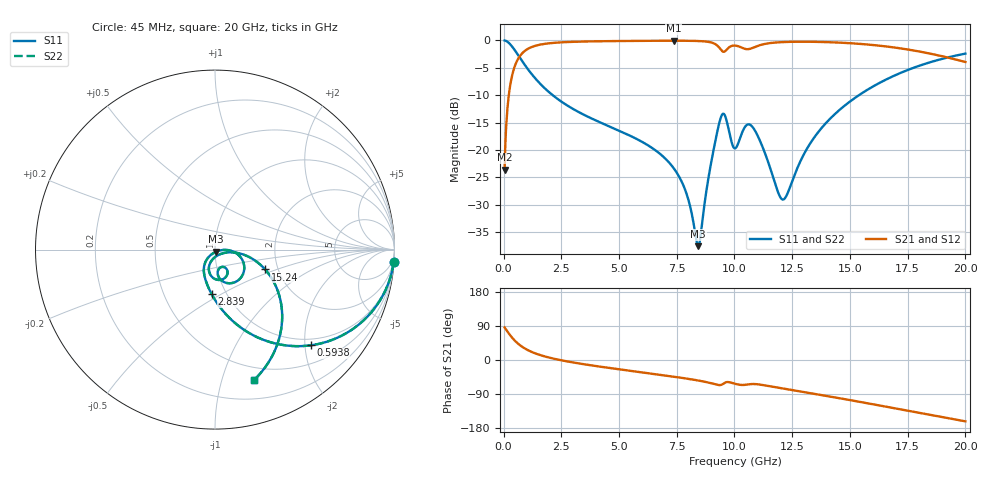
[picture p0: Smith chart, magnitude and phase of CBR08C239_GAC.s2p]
! S-parameter model data by Modelithics Inc.  support@modelithics.com 813-866-6335  Tampa FL USA
! S-Parameter data specifications:
! Substrate: 20-mil Rogers 4350B, substrate thickness, H=0.508mm, Dielectric constant, Er=3.75
! PCB Mounting Pad Footprint: Pad width, PadW=1.45mm , Pad length, PadL=1mm , Pad gap, PadG (edge-to-edge)=0.6mm , Reference planes=2.6mm apart
#  GHz  S  MA  R 50
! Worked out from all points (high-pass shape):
!   801 points, 45 MHz to 20 GHz, reference 50 ohm
!   highest |S21| = -0.07 dB at 7.378 GHz (marker M1); lowest = -23.6 dB at 45 MHz (marker M2)
!   |S21| within 3 dB of the highest: 674.3 MHz to 19.17 GHz (18.5 GHz wide, 186 % of centre)
!   lowest |S11| = -37.5 dB at 8.426 GHz (marker M3), VSWR 1.03, Z = 50.5 - j1.24 ohm
!   |S11| at or under -10 dB: 2.128 GHz to 15.39 GHz (13.26 GHz wide, 151 % of centre)
!   |S22| runs from -37.5 to 0.0 dB; largest |S21 - S12| = 0
!   S11 on the Smith chart (normalised r, x): 45 MHz: 1, -28; 593.8 MHz: 0.86, -2.12; 2.839 GHz: 0.85, -0.45; 15.24 GHz: 1.71, -0.42; 20 GHz: 0.38, -1.28
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0.045  0.9978 -4.1  0.06614 85.9  0.06614 85.9  0.9978 -4.1
0.269494  0.9294 -23.5  0.3687 66.5  0.3687 66.5  0.9294 -23.5
0.593762  0.7537 -45.1  0.6566 44.9  0.6566 44.9  0.7537 -45.1
1.391962  0.4453 -72.8  0.8941 17.1  0.8941 17.1  0.4453 -72.8
2.8387  0.2487 -94.3  0.9667 -4.6  0.9667 -4.6  0.2487 -94.3
3.387462  0.2145 -99.8  0.9747 -10.3  0.9747 -10.3  0.2145 -99.8
6.704981  0.09485 -126.4  0.9914 -38.4  0.9914 -38.4  0.09485 -126.4
7.378463  0.06776 -130.1  0.9922 -44.1  0.9922 -44.1  0.06776 -130.1
7.927225  0.03974 -128.6  0.9912 -49.0  0.9912 -49.0  0.03974 -128.6
8.4261  0.01329 -67.7  0.9862 -54.1  0.9862 -54.1  0.01329 -67.7
8.999806  0.07879 -2.8  0.9558 -61.5  0.9558 -61.5  0.07879 -2.8
9.42385  0.2019 -37.2  0.8166 -65.6  0.8166 -65.6  0.2019 -37.2
9.598456  0.2036 -67.2  0.7969 -59.5  0.7969 -59.5  0.2036 -67.2
10.0225  0.1036 -70.0  0.8961 -62.7  0.8961 -62.7  0.1036 -70.0
10.49643  0.1667 -70.5  0.8328 -65.3  0.8328 -65.3  0.1667 -70.5
10.77081  0.1633 -90.6  0.8508 -63.4  0.8508 -63.4  0.1633 -90.6
12.09283  0.03535 -62.8  0.9643 -75.3  0.9643 -75.3  0.03535 -62.8
13.36496  0.1224 -8.4  0.9702 -88.4  0.9702 -88.4  0.1224 -8.4
15.23574  0.3006 -21.6  0.9352 -108.3  0.9352 -108.3  0.3006 -21.6
16.68248  0.4516 -36.7  0.8739 -124.6  0.8739 -124.6  0.4516 -36.7
18.30382  0.6156 -54.7  0.7695 -143.2  0.7695 -143.2  0.6156 -54.7
20  0.757 -73.1  0.6345 -161.9  0.6345 -161.9  0.757 -73.1
